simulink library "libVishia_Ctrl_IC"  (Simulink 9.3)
settings: Solver=ode45  StartTime=0.0  StopTime=10.0  RelTol=1e-3  EnableMultiTasking=on
undefined symbols (not defined in the file or in its folder): TstepClk
libraries: libVishia_Ctrl x1

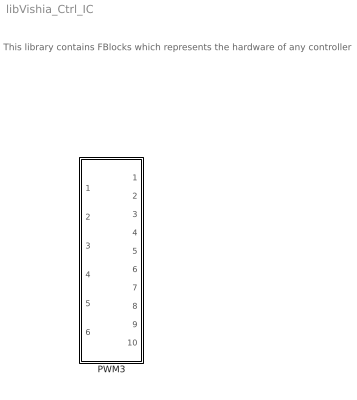
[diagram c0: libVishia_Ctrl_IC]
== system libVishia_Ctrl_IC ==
  note: This library contains FBlocks which represents the hardware of any controller
  PWM3 : Subsystem

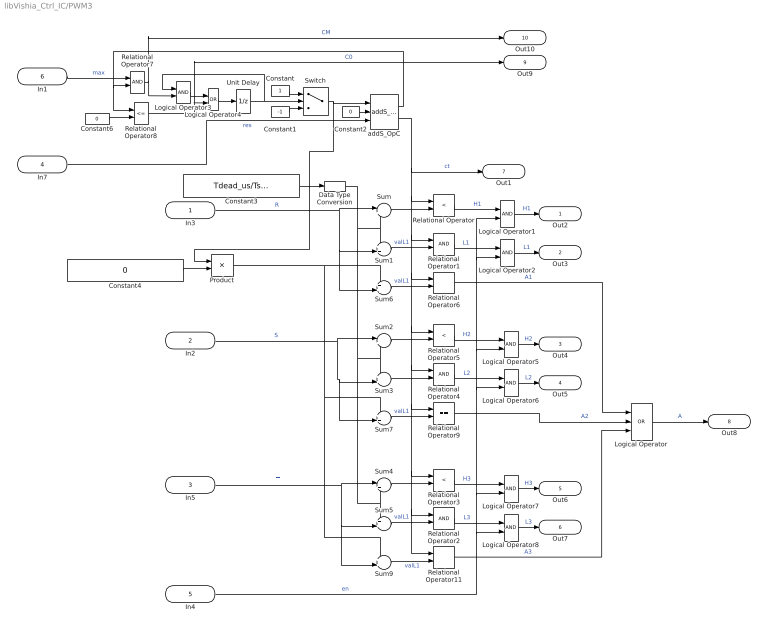
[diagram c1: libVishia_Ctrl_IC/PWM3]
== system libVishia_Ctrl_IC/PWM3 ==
  In3 : Inport  OutDataTypeStr=uint16
  In2 : Inport  Port=2  OutDataTypeStr=uint16
  In5 : Inport  Port=3  OutDataTypeStr=uint16
  In7 : Inport  Port=4  OutDataTypeStr=boolean
  In4 : Inport  Port=5  OutDataTypeStr=boolean
  In1 : Inport  Port=6  OutDataTypeStr=uint16
  Constant : Constant  OutDataTypeStr=int16
  Constant1 : Constant  Value=-1  OutDataTypeStr=int16
  Constant2 : Constant  Value=0  OutDataTypeStr=int16
  Constant3 : Constant  Value=Tdead_us/TstepClk/2000000  OutDataTypeStr=int16
  Constant4 : Constant  Value=0  OutDataTypeStr=int16
  Constant6 : Constant  Value=0  OutDataTypeStr=int16
  Data Type Conversion : DataTypeConversion  OutDataTypeStr=int16
  Logical Operator : Logic  Operator=OR  Inputs=3  IconShape=distinctive  AllPortsSameDT=off  OutDataTypeStr=boolean
  Logical Operator{1..2,5..8} (6 alike) : Logic  IconShape=distinctive  AllPortsSameDT=off  OutDataTypeStr=boolean
  Logical Operator3 : Logic  AllPortsSameDT=off  OutDataTypeStr=boolean
  Logical Operator4 : Logic  Operator=OR  AllPortsSameDT=off  OutDataTypeStr=boolean
  Product : Product
  Relational Operator : RelationalOperator  Operator=<  OutDataTypeStr=boolean  RndMeth=Simplest
  Relational Operator{1..2,4,7} (4 alike) : RelationalOperator  OutDataTypeStr=boolean  RndMeth=Simplest
  Relational Operator11 : RelationalOperator  Operator===  OutDataTypeStr=boolean  RndMeth=Simplest
  Relational Operator3 : RelationalOperator  Operator=<  OutDataTypeStr=boolean  RndMeth=Simplest
  Relational Operator5 : RelationalOperator  Operator=<  OutDataTypeStr=boolean  RndMeth=Simplest
  Relational Operator6 : RelationalOperator  Operator===  OutDataTypeStr=boolean  RndMeth=Simplest
  Relational Operator8 : RelationalOperator  Operator=<=  OutDataTypeStr=boolean  RndMeth=Simplest
  Relational Operator9 : RelationalOperator  Operator===  OutDataTypeStr=boolean  RndMeth=Simplest
  Sum : Sum  Inputs=|+-
  Sum{1,3,5..7,9} (6 alike) : Sum  Inputs=++|
  Sum2 : Sum  Inputs=|+-
  Sum4 : Sum  Inputs=|+-
  Switch : Switch  Criteria=u2 ~= 0
  Unit Delay : UnitDelay  InitialCondition=true  SampleTime=TstepClk  HasFrameUpgradeWarning=on
  addS_OpC : libVishia_Ctrl/addS_OpC  init=0  Tstep=-1
  Out2 : Outport  OutDataTypeStr=boolean
  Out3 : Outport  Port=2  OutDataTypeStr=boolean
  Out4 : Outport  Port=3  OutDataTypeStr=boolean
  Out5 : Outport  Port=4  OutDataTypeStr=boolean
  Out6 : Outport  Port=5  OutDataTypeStr=boolean
  Out7 : Outport  Port=6  OutDataTypeStr=boolean
  Out1 : Outport  Port=7  OutDataTypeStr=int16
  Out8 : Outport  Port=8  OutDataTypeStr=boolean
  Out9 : Outport  Port=9  OutDataTypeStr=boolean
  Out10 : Outport  Port=10  OutDataTypeStr=boolean
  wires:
  Switch/1 -> Product/1, addS_OpC/1
  Constant1/1 -> Switch/3
  Sum1/1 -> Relational Operator1/2  "valL1"
  In3/1 -> Sum6/2, Sum1/2, Sum/1  "R"
  Constant/1 -> Switch/1
  Logical Operator1/1 -> Out2/1  "H1"
  Logical Operator2/1 -> Out3/1  "L1"
  Logical Operator5/1 -> Out4/1  "H2"
  Logical Operator6/1 -> Out5/1  "L2"
  Logical Operator7/1 -> Out6/1  "H3"
  Logical Operator8/1 -> Out7/1  "L3"
  In7/1 -> addS_OpC/3  "res"
  Constant2/1 -> addS_OpC/2
  Sum/1 -> Relational Operator/2
  Constant3/1 -> Data Type Conversion/1
  Relational Operator8/1 -> Out9/1, Logical Operator4/2  "C0"
  Unit Delay/1 -> Switch/2, Logical Operator3/1
  Relational Operator7/1 -> Out10/1, Logical Operator3/2  "CM"
  addS_OpC/1 -> Relational Operator8/1, Relational Operator7/2
  Logical Operator3/1 -> Logical Operator4/1
  Logical Operator4/1 -> Unit Delay/1
  Constant6/1 -> Relational Operator8/2
  In1/1 -> Relational Operator7/1  "max"
  In2/1 -> Sum7/2, Sum3/2, Sum2/1  "S"
  Sum3/1 -> Relational Operator4/2
  Sum2/1 -> Relational Operator5/2
  In5/1 -> Sum4/1, Sum9/2, Sum5/2  "T"
  Sum5/1 -> Relational Operator2/2  "valL1"
  Sum4/1 -> Relational Operator3/2
  Sum6/1 -> Relational Operator6/2  "valL1"
  Logical Operator/1 -> Out8/1  "A"
  Constant4/1 -> Product/2
  Product/1 -> Sum9/1, Sum7/1, Sum6/1
  Sum7/1 -> Relational Operator9/2  "valL1"
  addS_OpC/2 -> Out1/1, Relational Operator/1, Relational Operator1/1, Relational Operator6/1, Relational Operator5/1, Relational Operator4/1, Relational Operator9/1, Relational Operator3/1, Relational Operator2/1, Relational Operator11/1  "ct"
  Data Type Conversion/1 -> Sum5/1, Sum4/2, Sum3/1, Sum2/2, Sum1/1, Sum/2
  Relational Operator9/1 -> Logical Operator/2  "A2"
  Relational Operator11/1 -> Logical Operator/3  "A3"
  Sum9/1 -> Relational Operator11/2  "valL1"
  Relational Operator6/1 -> Logical Operator/1  "A1"
  Relational Operator/1 -> Logical Operator1/1  "H1"
  Relational Operator1/1 -> Logical Operator2/1  "L1"
  Relational Operator5/1 -> Logical Operator5/1  "H2"
  Relational Operator4/1 -> Logical Operator6/1  "L2"
  Relational Operator3/1 -> Logical Operator7/1  "H3"
  Relational Operator2/1 -> Logical Operator8/1  "L3"
  In4/1 -> Logical Operator1/2, Logical Operator2/2, Logical Operator5/2, Logical Operator6/2, Logical Operator7/2, Logical Operator8/2  "en"
